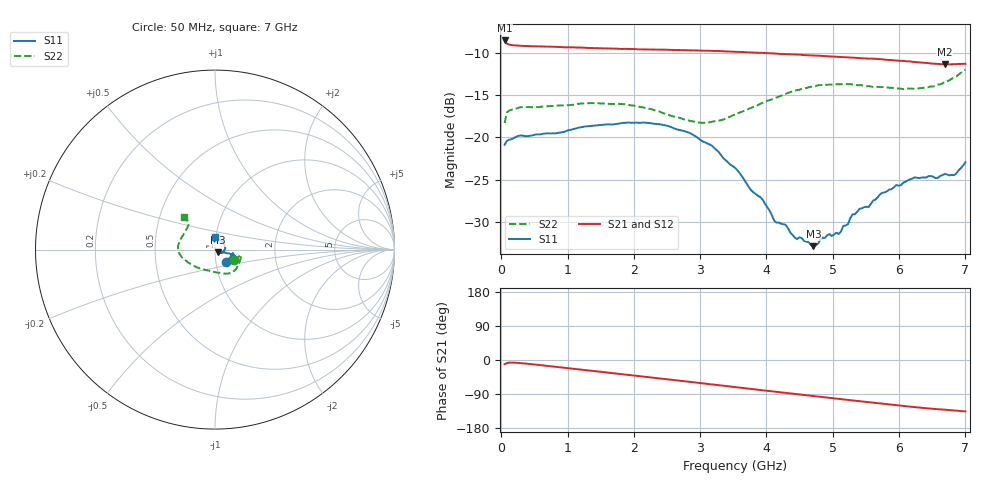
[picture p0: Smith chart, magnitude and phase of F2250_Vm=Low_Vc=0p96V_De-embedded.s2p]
! Integrated Device Technology
! Corporate Headquarters
! 6024 Silver Creek Valley Road
! San Jose, CA 95138  USA
! Phone:  1-408-284-8200
! Toll Free:  1-800-223-1366
! Webpage:  http://www.idt.com/
! Timing and RF Division
! 515 Groton Road, Suite 102
! Westford, MA 01886-6024
! Device:  F2250
! Description: Voltage Variable RF Attenuator
! Frequency:  50.0 -  6000.00 MHz
! Package:  3x3 mm Thin QFN Plastic Package: 16 pin
! Ports:  2 RF, 3 DC
!  Pin  1  = GND
!  Pin  2  = NC
!  Pin  3  = RF1  = Port 1
!  Pin  4  = NC
!  Pin  5  = GND
!  Pin  6  = GND
!  Pin  7  = GND
!  Pin  8  = GND
!  Pin  9  = NC
!  Pin 10  = RF2  = Port 2
!  Pin 11  = NC
!  Pin 12  = GND
!  Pin 13  = GND
!  Pin 14  = VCNTRL
!  Pin 15  = VDD
!  Pin 16  = VMODE
! Vcntrl:  0.960 Volts
! Vmode:  +0.000 Volts
! Vdd:  +3.30  Volts
! Current:  1.183 mA
! Data:  The device was measured on a the F2250 evaluation board which has
!  individual transmission lines to the RF pins.  Data was collected
!  using a calibrated network analyzer.  The evaluation board was
!  de-embedded using a TRL calibration technique.
!  The reference plane is the edge of the package pin.
! Misc:  SN 10
!  Action Tracker AT0258
! Date Measured:  2014-11-26
! Date:  2015-10-15  MJV
! Note:
!  Integrated Device Technology supplies this data as a sample of measured
!  data at the package pin for this product.  Your particular data for this
!  product may vary.
!  Data was taken at 25 degrees C.
!  Integrated Device Technology reserves the right to change this data at anytime.
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# GHz S dB R 50
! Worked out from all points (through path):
!   201 points, 50 MHz to 7 GHz, reference 50 ohm
!   highest |S21| = -8.52 dB at 50 MHz (marker M1); lowest = -11.3 dB at 6.687 GHz (marker M2)
!   group delay of S21, straight-line fit = 54.1 ps
!   lowest |S11| = -32.9 dB at 4.707 GHz (marker M3), VSWR 1.05, Z = 51.6 - j1.64 ohm
!   |S11| at or under -10 dB: start of sweep to end of sweep
!   |S22| runs from -18.3 to -12.0 dB; largest |S21 - S12| = 0.0009
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0.05  -20.86 -48.6  -8.52 -10.9  -8.52 -10.9  -18.29 -28.4
0.08475  -20.39 -25.6  -8.89 -8.0  -8.90 -8.0  -17.03 -15.5
0.29325  -19.76 -11.1  -9.15 -8.2  -9.15 -8.2  -16.42 -14.0
1.2315  -18.75 -21.2  -9.38 -26.0  -9.38 -26.0  -15.96 -41.9
1.857  -18.27 -21.4  -9.51 -38.1  -9.51 -38.1  -16.06 -56.1
2.37825  -18.42 -18.9  -9.60 -48.3  -9.60 -48.3  -16.91 -69.7
3.0385  -20.47 -15.6  -9.74 -61.6  -9.72 -61.6  -18.27 -101.5
3.525  -23.58 -17.4  -9.86 -71.5  -9.86 -71.5  -17.27 -131.0
3.76825  -26.24 -20.0  -9.94 -76.4  -9.94 -76.4  -16.49 -143.1
3.942  -27.36 -23.4  -9.99 -79.9  -10.00 -79.9  -15.90 -150.9
4.11575  -29.84 -27.7  -10.06 -83.4  -10.07 -83.4  -15.37 -157.8
4.4285  -31.85 -38.7  -10.18 -89.7  -10.19 -89.6  -14.44 -167.1
4.7065  -32.87 -44.4  -10.31 -95.2  -10.30 -95.2  -13.98 -174.0
4.94975  -31.43 -41.9  -10.41 -100.0  -10.41 -100.0  -13.74 -179.3
5.08875  -31.42 -37.7  -10.46 -102.7  -10.46 -102.7  -13.71 177.5
5.29725  -29.10 -31.1  -10.54 -106.7  -10.54 -106.8  -13.71 172.9
5.5405  -28.24 -20.2  -10.67 -111.4  -10.66 -111.4  -13.92 166.6
5.85325  -26.17 -9.8  -10.82 -117.3  -10.82 -117.4  -14.11 158.5
6.2355  -24.72 10.4  -11.07 -124.3  -11.07 -124.3  -14.23 145.9
6.68725  -24.33 48.7  -11.35 -131.1  -11.35 -131.1  -13.43 134.2
6.82625  -24.46 64.3  -11.31 -133.1  -11.32 -133.1  -12.92 134.0
7  -22.92 89.8  -11.28 -135.7  -11.29 -135.8  -11.98 133.8
